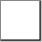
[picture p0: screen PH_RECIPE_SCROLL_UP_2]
VISUALIZATION PH_RECIPE_SCROLL_UP_2  // 42x42
VAR_IN_OUT
	RECIPE_CTRL_V2 : None;
END_VAR
    Rectangle (0,0 40x40)
        tap RECIPE_CTRL_V2.sCmd.bScrollUp
    Polygon (20,10), colour toggle: (RECIPE_CTRL_V2.sCmd.bScrollUp) <> 0
        tap RECIPE_CTRL_V2.sCmd.bScrollUp
END_VISUALIZATION
